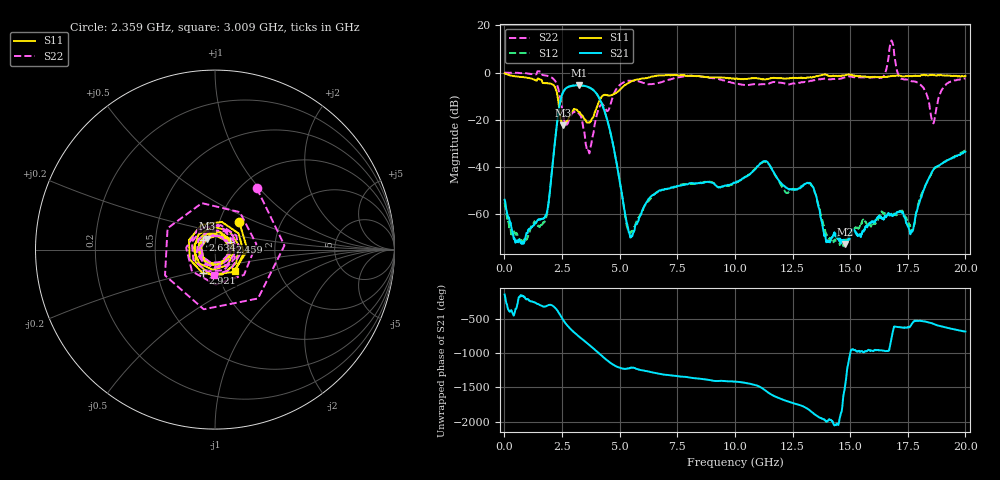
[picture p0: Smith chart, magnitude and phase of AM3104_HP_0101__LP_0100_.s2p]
!Created with skrf (http://scikit-rf.org).
# Hz S RI R 50.0
!freq ReS11 ImS11 ReS21 ImS21 ReS12 ImS12 ReS22 ImS22
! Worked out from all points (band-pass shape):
!   1601 points, 10 MHz to 20 GHz, reference 50 ohm
!   highest |S21| = -5.36 dB at 3.233 GHz (marker M1); lowest = -72.8 dB at 14.78 GHz (marker M2)
!   |S21| within 3 dB of the highest: 2.544 GHz to 3.951 GHz (1.407 GHz wide, 43.3 % of centre)
!   lowest |S11| = -22.4 dB at 2.534 GHz (marker M3), VSWR 1.16, Z = 45.3 + j5.49 ohm
!   |S11| at or under -10 dB: 2.306 GHz to 4.244 GHz (1.937 GHz wide, 59.2 % of centre)
!   |S22| runs from -34.3 to 13.6 dB; largest |S21 - S12| = 0.029
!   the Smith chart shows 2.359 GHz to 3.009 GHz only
!   S11 on the Smith chart (normalised r, x): 2.359 GHz: 1.24, +0.40; 2.459 GHz: 1.18, +0.11; 2.634 GHz: 0.87, +0.09; 2.921 GHz: 0.84, -0.23; 3.009 GHz: 1.21, -0.30
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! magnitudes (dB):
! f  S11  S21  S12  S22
! 10 MHz  -0.3  -54.0  -55.1  0.0
! 509.8 MHz  -1.6  -71.7  -68.1  -0.1
! 1.697 GHz  -4.5  -62.1  -63.8  -1.1
! 2.359 GHz  -13.7  -15.9  -16.0  -7.7
! 2.459 GHz  -20.3  -10.8  -10.8  -12.7
! 2.534 GHz  -22.4  -8.6  -8.6  -17.3
! 2.634 GHz  -21.2  -7.0  -7.0  -21.8
! 2.921 GHz  -16.6  -5.6  -5.7  -17.5
! 3.009 GHz  -15.7  -5.5  -5.5  -16.9
! 3.233 GHz  -16.8  -5.4  -5.5  -17.4
! 3.346 GHz  -17.9  -5.5  -5.5  -19.3
! 3.658 GHz  -21.1  -6.2  -6.3  -33.4
! 4.358 GHz  -9.4  -16.7  -16.7  -15.0
! 5.47 GHz  -4.0  -70.0  -68.1  -3.5
! 6.682 GHz  -1.2  -50.4  -50.4  -4.5
! 10.01 GHz  -2.7  -46.8  -47.1  -4.6
! 13.34 GHz  -2.1  -47.9  -48.0  -3.5
! 14.78 GHz  -1.1  -72.8  -71.8  -2.0
! 16.68 GHz  -1.6  -59.9  -60.4  7.2
! 17.66 GHz  -1.5  -67.7  -67.4  -3.7
! 18.59 GHz  -1.0  -41.6  -41.9  -21.1
! 20 GHz  -1.5  -33.6  -33.1  -2.5
